TYPE CKD_IN :
STRUCT
	WcStateOut	:	BIT	;		
	Value_Sensor_Input1	:	REAL	;	//	Value sensor input1 (p1)
	Value_Sensor_Input2	:	REAL	;	//	Value sensor input2 (p2)
	Position_Actual_Value	:	REAL	;	//	Position actual value 
	Control_Mode_Status	:	USINT	;//	"Control mode status:
									(*	Indicates the current controlmode.
									O: IDLE
									1:HOMING(Auto teaching)
									2: POS(Valve Opening Control
									3: Reserved
									4: HOID(Valve Opening Hld)
									5:CLOSE(Close)
									6:OPEN(Open
									7:PRESS1(P1 SensorVacuum Pessure Control
									8:PRESS2(P2 SensorVacuum Pressure Control
									9 to 15: Reserved
									16:SIOWVAC(Sow Vacuum Control"
									*)	
	Homing_Status	:	USINT	;	//	"HOME status
									(*
									indicates the homing status.
									0: Homing not started
									1: Homing interrupted
									2: Homing completed-no error
									3:Homing completed-error204: Hmingin progress
									5to 255: Reserved"
									*)
	
	Selected_Controller	:	USINT	;	//	"Select controller
											(*
											Indicates The PIDtables used.
											1: 0x8060(rocess Controller 1)
											2:0x8070(Pocess Cntroller2)
											3:0x8080(cess Cntroller3)
											4:0x8090(Process Cntroller 4)
											5:0x80A0(Process Controller5)
											6:0x80M(Pocess ntroller6
											7:0x80C0(Process Controller 7
											8:0x80D0(Process Cntroller8
											9:0x80E(Pocess Controller 9)
											10: 0x80F(Pocess Controller 10)
											11: 0x5050(SVA0"
											*)
	Device_Management_Device_Warning_Details	:	UDINT	;	//	Active Device Warning Details (Device Management)
	Sensor_Input1_Device_Warning_Details	:	UDINT	;	//	Active Device Warning Details (Sensor put1)
	Sensor_Input2_Device_Warning_Details	:	UDINT	;	//	Active Device Warning Details (Sensor Input2)
	Process_Controller_Selector_Device_Warning_Details	:	UDINT	;	//	Active Device Warning Details (Process Controller Selector)
	Valve_Device_Warning_Details	:	UDINT	;	//	Active Device Warning Details (Valve)
	Valve_manufacturer_Warning_Details	:	UDINT	;	//	Active manufacturer Warning Details (Valve)
	Device_Management_manufacturer_Error_Details	:	UDINT	;	//	Active manufacturer Error Details (Device Management)
	Sensor_Input1_Management_manufacturer_Error_Details	:	UDINT	;	//	Active manufacturer Error Details(Sensor Input1)
	Sensor_Input2_Management_manufacturer_Error_Details	:	UDINT	;	//	Active manufacturer Error Details (Sensor Input2)
	Valve_Management_manufacturer_Error_Details	:	UDINT	;	//	Active manufacturer Error Details (Valve)
	WcStateIn	:	BIT	;	//	
	InputToggle	:	BIT	;	//	
	State	:	UINT	;	//	

END_STRUCT
END_TYPE
